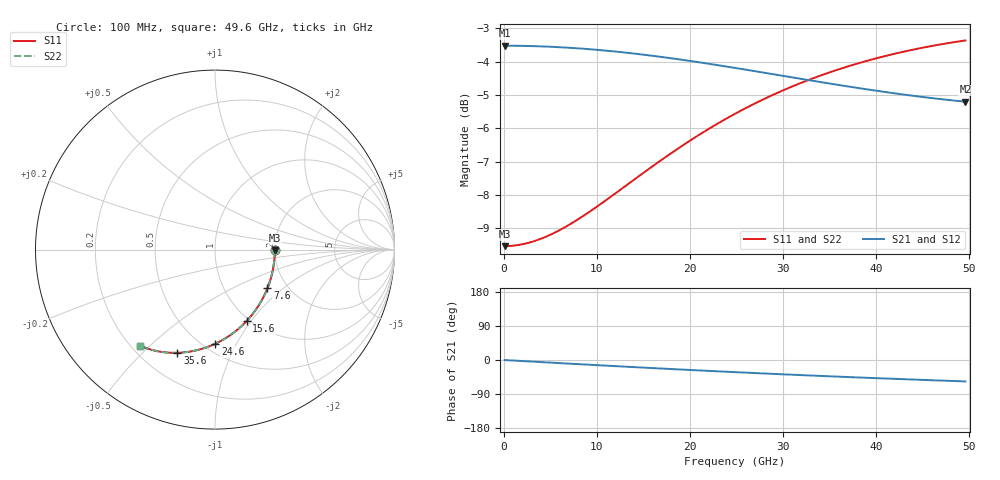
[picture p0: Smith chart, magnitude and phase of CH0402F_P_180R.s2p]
# GHz S RI R 180
! S-Parameters data
! Freq  reS11  imS11  reS21  imS21  reS12  imS12  reS22  imS22
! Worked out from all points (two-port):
!   100 points, 100 MHz to 49.6 GHz, reference 180 ohm
!   highest |S21| = -3.52 dB at 100 MHz (marker M1); lowest = -5.2 dB at 49.6 GHz (marker M2)
!   |S21| within 3 dB of the highest: start of sweep to end of sweep
!   lowest |S11| = -9.5 dB at 100 MHz (marker M3), VSWR 2.00, Z = 360 - j2.37 ohm
!   |S11| at or under -10 dB: nowhere
!   |S22| runs from -9.5 to -3.4 dB; largest |S21 - S12| = 0
!   S11 on the Smith chart (normalised r, x): 100 MHz: 2.00, -0.01; 7.6 GHz: 1.59, -0.79; 15.6 GHz: 0.97, -0.95; 24.6 GHz: 0.57, -0.82; 35.6 GHz: 0.35, -0.64; 49.6 GHz: 0.23, -0.47
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0.1  0.3333 -0.00293  0.6667 -0.00159  0.6667 -0.00159  0.3333 -0.00293
1.6  0.3315 -0.0468  0.6659 -0.0254  0.6659 -0.0254  0.3315 -0.0468
3.6  0.3239 -0.1047  0.663 -0.057  0.663 -0.057  0.3239 -0.1047
5.6  0.3106 -0.1612  0.6578 -0.0882  0.6578 -0.0882  0.3106 -0.1612
7.6  0.2922 -0.2153  0.6504 -0.1186  0.6504 -0.1186  0.2922 -0.2153
8.6  0.2811 -0.2414  0.646 -0.1335  0.646 -0.1335  0.2811 -0.2414
12.1  0.2338 -0.3259  0.6268 -0.1834  0.6268 -0.1834  0.2338 -0.3259
15.6  0.1758 -0.3984  0.6027 -0.2292  0.6027 -0.2292  0.1758 -0.3984
16.6  0.1578 -0.4167  0.5951 -0.2415  0.5951 -0.2415  0.1578 -0.4167
18.6  0.1203 -0.4501  0.5789 -0.2648  0.5789 -0.2648  0.1203 -0.4501
20.6  0.0814 -0.4791  0.5618 -0.2866  0.5618 -0.2866  0.0814 -0.4791
22.6  0.0416 -0.5038  0.544 -0.3067  0.544 -0.3067  0.0416 -0.5038
24.6  0.00148 -0.5245  0.5257 -0.3253  0.5257 -0.3253  0.00148 -0.5245
25.1  -0.00855 -0.529  0.521 -0.3297  0.521 -0.3297  -0.00855 -0.529
27.1  -0.0485 -0.5448  0.5023 -0.3463  0.5023 -0.3463  -0.0485 -0.5448
29.1  -0.088 -0.557  0.4834 -0.3615  0.4834 -0.3615  -0.088 -0.557
33.1  -0.1641 -0.5716  0.4457 -0.3879  0.4457 -0.3879  -0.1641 -0.5716
35.6  -0.2092 -0.575  0.4225 -0.402  0.4225 -0.402  -0.2092 -0.575
38.6  -0.2604 -0.574  0.3953 -0.4169  0.3953 -0.4169  -0.2604 -0.574
41.6  -0.3081 -0.5682  0.3689 -0.4299  0.3689 -0.4299  -0.3081 -0.5682
45.6  -0.3661 -0.5546  0.3352 -0.445  0.3352 -0.445  -0.3661 -0.5546
49.6  -0.4176 -0.5353  0.3031 -0.4582  0.3031 -0.4582  -0.4176 -0.5353
